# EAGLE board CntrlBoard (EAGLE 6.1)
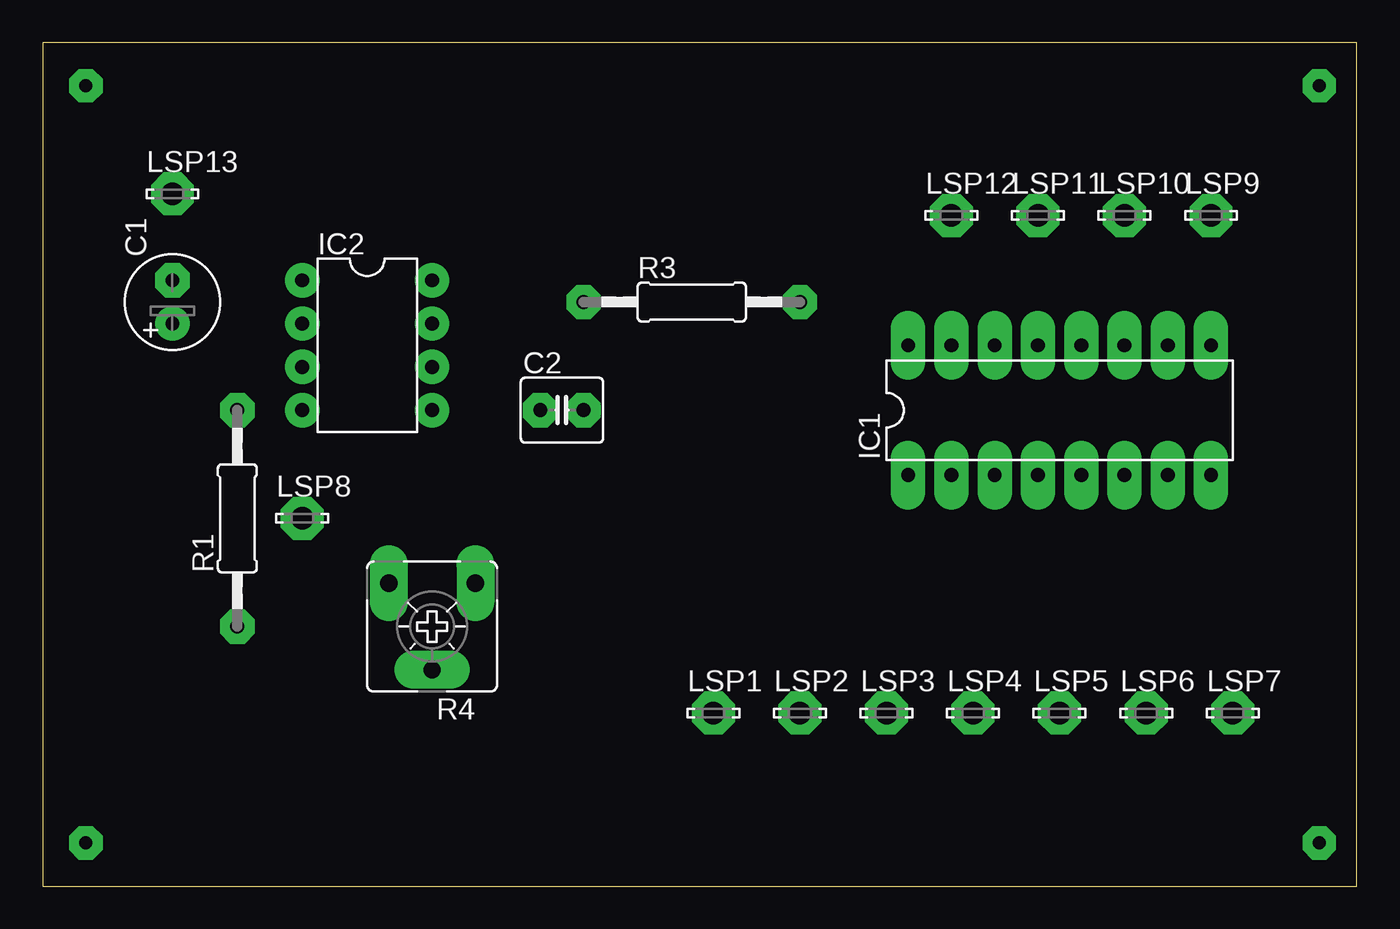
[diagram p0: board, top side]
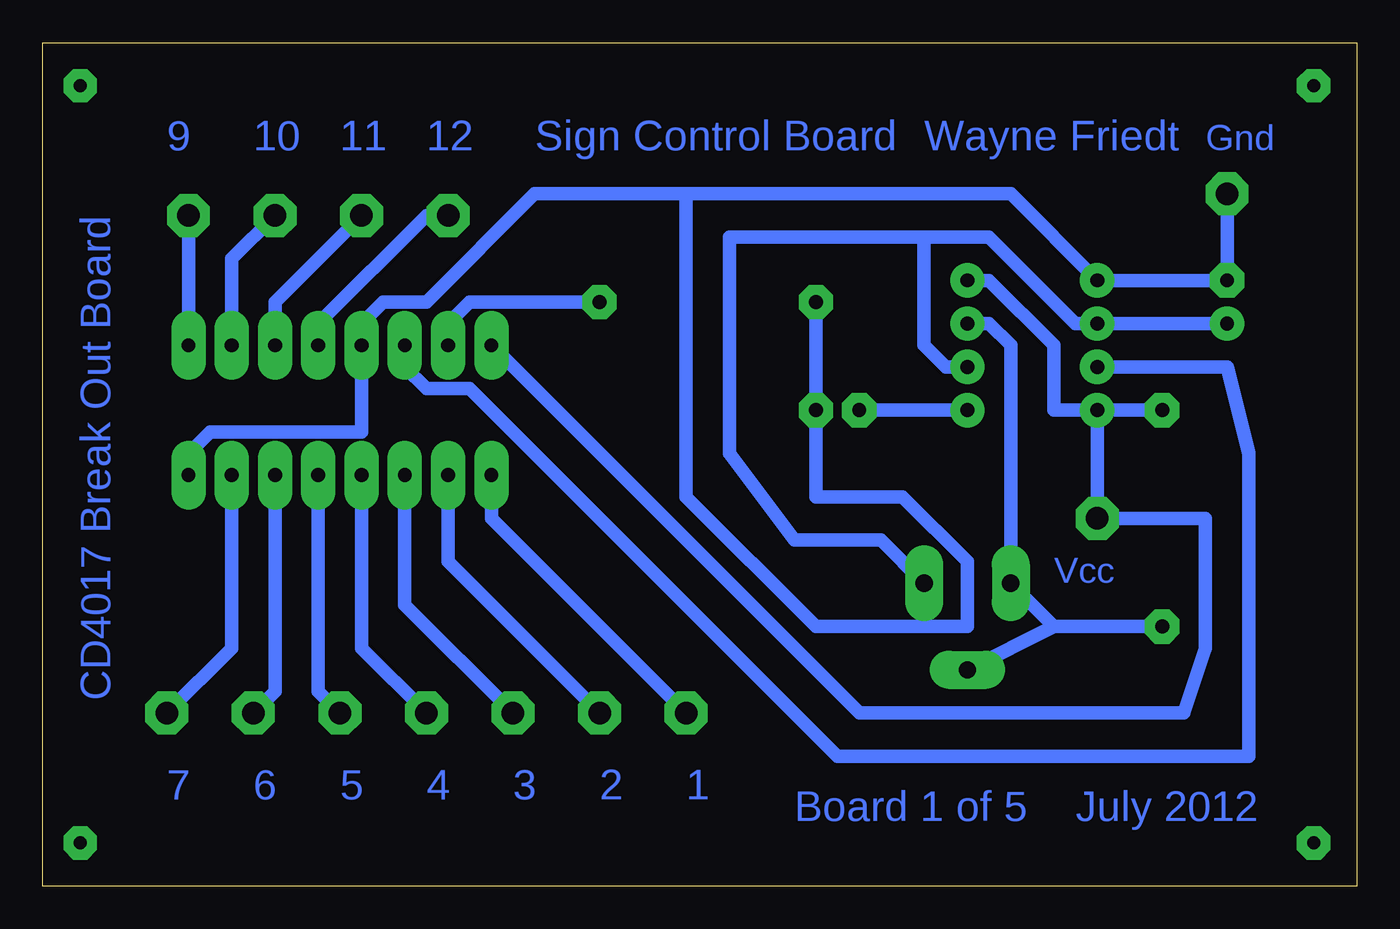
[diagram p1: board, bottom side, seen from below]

Size 77.14 x 49.52 mm. Coordinates in mm from the lower left corner, seen from the top.
Outline: 0,0 77.14,0 77.14,49.52 0,49.52 0,0
Copper layers (1*16): Top 0.035mm / dielectric 1.5mm / Bottom 0.035mm
Design rules: minimum track width 0.8mm, minimum drill 0.8mm, track to track 0.8mm, track to pad 0.8mm, pad to pad 0.45mm, via to via 0.8mm, smd to smd 8mil, copper to edge 10mil, drill to drill 8mil, minimum pad ring 0.6mm, minimum via ring 0.6mm, stop-mask expansion 0mil, vias tented up to drill 0mil, thermal gap 10mil

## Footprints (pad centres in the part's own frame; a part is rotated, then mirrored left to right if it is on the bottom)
E2,5-6 = drill 0.813 pad 1.6: + -1.27,0 | drill 0.813 pad 1.6 octagon: - 1.27,0
C025-040X050 = drill 0.813 octagon: 1 -1.27,0; 2 1.27,0
DIL16 = drill 0.813 long: 1 -8.89,-3.81; 2 -6.35,-3.81; 3 -3.81,-3.81; 4 -1.27,-3.81; 5 1.27,-3.81; 6 3.81,-3.81; 7 6.35,-3.81; 8 8.89,-3.81; 9 8.89,3.81; 10 6.35,3.81; 11 3.81,3.81; 12 1.27,3.81; 13 -1.27,3.81; 14 -3.81,3.81; 15 -6.35,3.81; 16 -8.89,3.81
DIL08 = drill 0.813 pad 1.27: 1 -3.81,-3.81; 2 -1.27,-3.81; 3 1.27,-3.81; 4 3.81,-3.81; 5 3.81,3.81; 6 1.27,3.81; 7 -1.27,3.81; 8 -3.81,3.81
LSP13 = drill 1.321 pad 2.159 octagon: MP 0,0
0207/12 = drill 0.813 octagon: 1 -6.35,0; 2 6.35,0
CA6V = drill 1.016 long: A -2.54,-2.54; E 2.54,-2.54; S 0,2.54

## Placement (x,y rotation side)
C1  10uF 16V  [E2,5-6]  7.62,34.29 90 top
C2  .01 uF  [C025-040X050]  30.48,27.94 0 top
IC1  4017N  [DIL16]  59.69,27.94 0 top
IC2  LM555N  [DIL08]  19.05,31.75 270 top
LSP1  LSP13  [LSP13]  39.37,10.16 0 top
LSP2  LSP13  [LSP13]  44.45,10.16 0 top
LSP3  LSP13  [LSP13]  49.53,10.16 0 top
LSP4  LSP13  [LSP13]  54.61,10.16 0 top
LSP5  LSP13  [LSP13]  59.69,10.16 0 top
LSP6  LSP13  [LSP13]  64.77,10.16 0 top
LSP7  LSP13  [LSP13]  69.85,10.16 0 top
LSP8  LSP13  [LSP13]  15.24,21.59 0 top
LSP9  LSP13  [LSP13]  68.58,39.37 0 top
LSP10  LSP13  [LSP13]  63.5,39.37 0 top
LSP11  LSP13  [LSP13]  58.42,39.37 0 top
LSP12  LSP13  [LSP13]  53.34,39.37 0 top
LSP13  LSP13  [LSP13]  7.62,40.64 0 top
R1  10K  [0207/12]  11.43,21.59 90 top
R3  10K  [0207/12]  38.1,34.29 0 top
R4  [CA6V]  22.86,15.24 180 top

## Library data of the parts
C1 C2 R1 R3 = resistor
IC1 = 40xx
IC2 = linear
LSP1-LSP13 = solpad
R4 = pot

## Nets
N$1: IC1.3 LSP3.MP
N$2: IC1.16 IC2.4 IC2.8 LSP8.MP R1.2
N$3: IC2.7 R1.1 R4.E R4.S
N$4: IC1.14 IC2.3
N$5: IC1.2 LSP2.MP
N$6: C2.1 IC2.5
N$7: IC1.4 LSP4.MP
N$8: IC1.7 LSP7.MP
N$9: C1.- C2.2 IC1.8 IC1.13 IC2.1 LSP13.MP R3.1
N$10: C1.+ IC2.2 IC2.6 R4.A
N$11: IC1.15 R3.2
N$12: IC1.10 LSP10.MP
N$13: IC1.1 LSP1.MP
N$14: IC1.5 LSP5.MP
N$15: IC1.6 LSP6.MP
N$16: IC1.9 LSP9.MP
N$17: IC1.11 LSP11.MP
N$18: IC1.12 LSP12.MP

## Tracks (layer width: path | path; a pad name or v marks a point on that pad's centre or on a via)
N$1
  Bottom 0.8: IC1.3 55.88,16.51 LSP3.MP
N$2
  Bottom 0.8: IC2.4 LSP8.MP 8.89,21.59 8.89,13.97 10.16,10.16 29.21,10.16 IC1.16 | IC2.4 R1.2 | IC2.8 21.59,35.56 17.78,31.75 17.78,27.94 IC2.4
N$3
  Bottom 0.8: IC2.7 21.59,33.02 20.32,31.75 R4.E 17.78,15.24 | 17.78,15.24 R1.1 | 17.78,15.24 R4.S
N$4
  Bottom 0.8: IC2.3 7.62,30.48 6.35,25.4 6.35,7.62 30.48,7.62 52.07,29.21 54.61,29.21 55.88,30.48 IC1.14
N$5
  Bottom 0.8: IC1.2 53.34,19.05 LSP2.MP
N$6
  Bottom 0.8: C2.1 IC2.5
N$7
  Bottom 0.8: IC1.4 58.42,13.97 LSP4.MP
N$8
  Bottom 0.8: IC1.7 66.04,13.97 LSP7.MP
N$9
  Bottom 0.8: LSP13.MP C1.- IC2.1 20.32,40.64 39.37,40.64 | R3.1 C2.2 31.75,22.86 26.67,22.86 22.86,19.05 22.86,15.24 31.75,15.24 39.37,22.86 39.37,40.64 | IC1.8 68.58,25.4 67.31,26.67 58.42,26.67 IC1.13 58.42,33.02 57.15,34.29 54.61,34.29 48.26,40.64 39.37,40.64
N$10
  Bottom 0.8: IC2.6 24.13,30.48 25.4,31.75 25.4,38.1 | 25.4,38.1 21.59,38.1 16.51,33.02 IC2.2 C1.+ | R4.A 27.94,20.32 33.02,20.32 36.83,25.4 36.83,38.1 25.4,38.1
N$11
  Bottom 0.8: R3.2 52.07,34.29 53.34,33.02 IC1.15
N$12
  Bottom 0.8: IC1.10 66.04,36.83 LSP10.MP
N$13
  Bottom 0.8: IC1.1 50.8,21.59 LSP1.MP
N$14
  Bottom 0.8: IC1.5 60.96,11.43 LSP5.MP
N$15
  Bottom 0.8: IC1.6 63.5,11.43 LSP6.MP
N$16
  Bottom 0.8: LSP9.MP IC1.9
N$17
  Bottom 0.8: IC1.11 63.5,34.29 LSP11.MP
N$18
  Bottom 0.8: IC1.12 60.96,33.02 54.61,39.37 LSP12.MP
S$1  (via drill 0.76)
  other vias: 2.54,2.54 2.54,46.99 74.93,46.99 74.93,2.54

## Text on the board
Bottom: Gnd | Wayne Friedt | Sign Control Board | 12 | 11 | 10 | 9 | CD4017 Break Out Board | Vcc | 1 | 2 | 3 | 4 | 5 | 6 | 7 | July 2012 | Board 1 of 5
